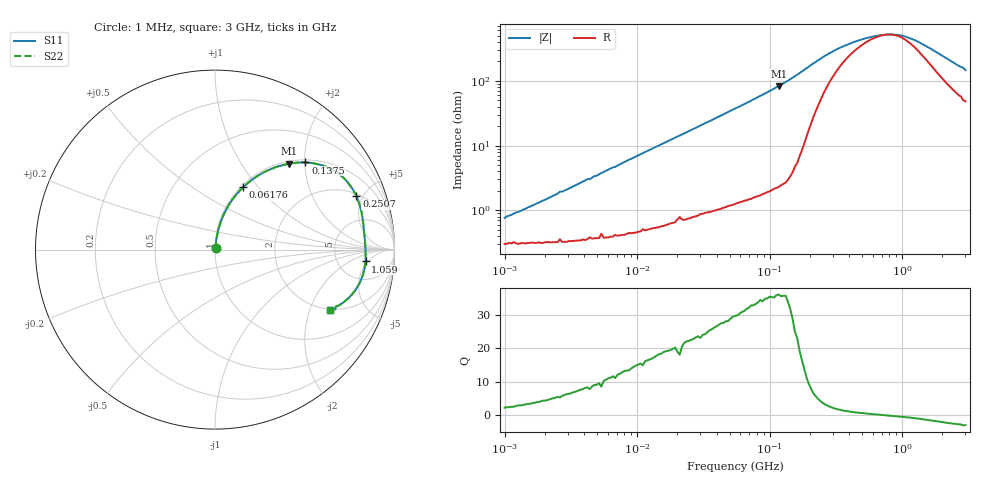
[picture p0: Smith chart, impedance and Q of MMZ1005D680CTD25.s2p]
! S-Parameter Data Generated by TDK Corporation
! Copyright(C) 2025 TDK Corporation.
! All Rights Reserved.
! TDK P/N: MMZ1005D680CTD25 (Chip Bead)
! Property: |Z|=68ohm at 100MHz
! Size(LxWxT): 1x0.5x0.5mm
! Model Type: s2p (Touchstone File Format Version 1.0)
! Frequency: DC=Yes Start=1MHz Stop=3000MHz 202points Log-sweep
! Model Generated on Feb. 6, 2025
! Terms and conditions regarding TDK Simulation Models:
! 1)This simulation model is being provided solely for informational
!  purposes. Please refer to the specifications of the products in
!  terms of detailed characteristics of such products.
! 2)In no event shall TDK Corporation of any of its subsidiaries be
!  liable for any loss or damage arising, directly or indirectly,
!  from any information contained in this simulation model, including,
!  but not limited to loss or damages arising from any inaccuracies,
!  omissions or errors in connection with such information.
! 3)Any and all copyrights on this simulation model are owned by
!  TDK Corporation.  Duplication or redistribution of this simulation
!  model without prior written permission from TDK Corporation
!  is prohibited.
! 4)This simulation model is subject to any modification or change
!  without any prior notice.
! 5)Neither TDK Corporation nor any of its subsidiaries shall make any
!  warranty, express or implied, including but not limited to the
!  correctness, implied warranties of merchantability and fitness for
!  a particular purpose with respect to this simulation models.
! 6)The use of this simulation model shall be deemed to have consented
!  to the terms and conditions hereof.
! Port Assignments:
!  1 ---@@@--- 2
! Applicable Conditions:
!  Temperature = 25 degC
!  DC Bias Current = 0 A
!  Small Signal Operation
# Hz S MA R 50
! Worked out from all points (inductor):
!   201 points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, 1 MHz to 3 GHz, reference 50 ohm
!   read as one part in series: L = 113 nH near 1.323 MHz
!   highest Q = 35.7 at 117.2 MHz (marker M1), where L = 113 nH
!   self-resonance near 784.5 MHz
!   S11 on the Smith chart (normalised r, x): 1 MHz: 1.01, +0.01; 61.76 MHz: 1.03, +0.84; 137.5 MHz: 1.06, +2.02; 250.7 MHz: 2.18, +4.46; 1.059 GHz: 10, -4; 3 GHz: 1.96, -2.76
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1000000  0.007582 66.2  0.997 -0.4  0.997 -0.4  0.007582 66.2
3900413  0.02781 81.1  0.9961 -1.6  0.9961 -1.6  0.02781 81.1
4398124  0.03009 81.0  0.9957 -1.7  0.9957 -1.7  0.03009 81.0
1.461624e7  0.09948 81.2  0.9896 -5.7  0.9896 -5.7  0.09948 81.2
3.127247e7  0.2058 75.8  0.9701 -11.9  0.9701 -11.9  0.2058 75.8
5.477226e7  0.3444 67.9  0.9273 -20.1  0.9273 -20.1  0.3444 67.9
6.176144e7  0.3825 65.7  0.9117 -22.5  0.9117 -22.5  0.3825 65.7
8.507507e7  0.4987 58.4  0.8525 -29.9  0.8525 -29.9  0.4987 58.4
1.171891e8  0.631 49.3  0.7585 -39.1  0.7585 -39.1  0.631 49.3
1.375402e8  0.6999 43.9  0.6939 -44.4  0.6939 -44.4  0.6999 43.9
1.680187e8  0.7774 36.1  0.5903 -50.9  0.5903 -50.9  0.7774 36.1
2.136344e8  0.8304 26.2  0.4472 -55.2  0.4472 -55.2  0.8304 26.2
2.507343e8  0.8423 20.6  0.3648 -54.5  0.3648 -54.5  0.8423 20.6
3.188066e8  0.8428 14.2  0.2758 -48.5  0.2758 -48.5  0.8428 14.2
4.391493e8  0.8376 8.2  0.2082 -34.9  0.2082 -34.9  0.8376 8.2
6.049187e8  0.8366 3.5  0.1728 -17.3  0.1728 -17.3  0.8366 3.5
8.005644e8  0.8388 -0.3  0.1613 1.5  0.1613 1.5  0.8388 -0.3
1.059487e9  0.8411 -4.5  0.1745 22.3  0.1745 22.3  0.8411 -4.5
1.294266e9  0.839 -7.9  0.2045 34.3  0.2045 34.3  0.839 -7.9
1.855641e9  0.8173 -15.4  0.3032 45.6  0.3032 45.6  0.8173 -15.4
2.882277e9  0.7484 -26.3  0.4678 45.2  0.4678 45.2  0.7484 -26.3
3e9  0.7223 -27.8  0.4936 43.0  0.4936 43.0  0.7223 -27.8
